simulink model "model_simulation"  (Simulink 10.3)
settings: Solver=VariableStepDiscrete  StartTime=0.0  StopTime=ts  RelTol=1e-3  EnableMultiTasking=on
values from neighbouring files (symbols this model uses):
  A = [0.9944 -0.1203 -0.4302    [model.m]
  Ao1 = A - K1*c1    [model.m]
  Ao2 = A - K2*c2    [model.m]
  Ao3 = A - K3*c3    [model.m]
  B = [0.4252 -0.0082 0.1813]'    [model.m]
  Bo1 = [B K1]    [model.m]
  Bo2 = [B K2]    [model.m]
  Bo3 = [B K3]    [model.m]
  C = eye(3)    [model.m]
  Co1 = c1    [model.m]
  Co2 = c2    [model.m]
  Co3 = c3    [model.m]
  D = zeros(3,1)    [model.m]
  Do1 = zeros(1,2)    [model.m]
  Do2 = zeros(1,2)    [model.m]
  Do3 = zeros(1,2)    [model.m]
  Tc = 0.1    [model.m]
  tf1 = ts/2    (= 25)    [model.m]
  tf2 = ts/2    (= 25)    [model.m]
  tf3 = ts/2    (= 25)    [model.m]
  x0 = [0.05 0.15 0.2]    [model.m]

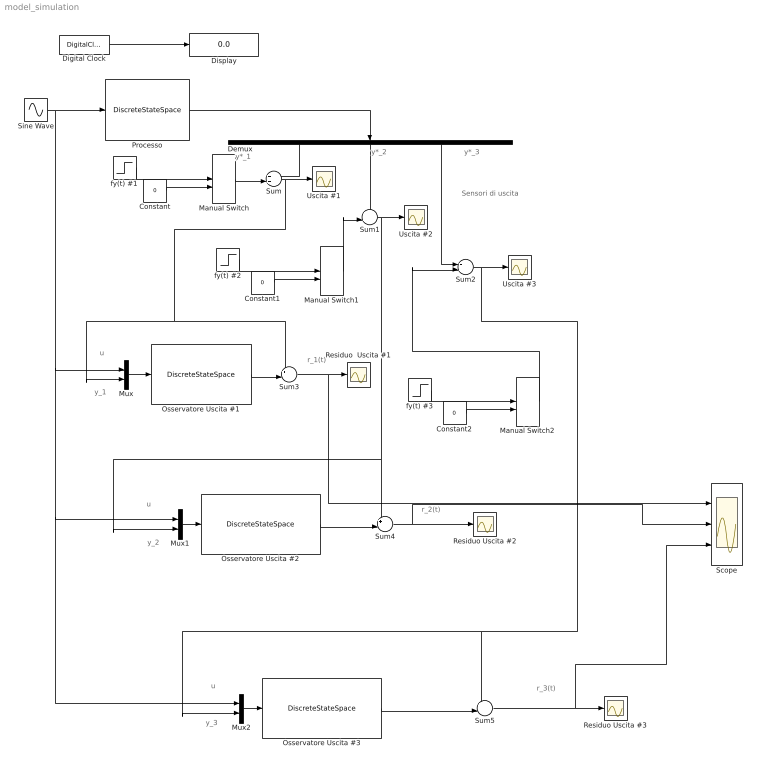
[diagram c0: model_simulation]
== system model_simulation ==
  note: Sensori di uscita
  note: y*_3
  note: y*_2
  note: y*_1
  note: u
  note: y_1
  note: u
  note: y_2
  note: u
  note: y_3
  note: r_1(t)
  note: r_2(t)
  note: r_3(t)
  Constant : Constant  Value=0
  Constant1 : Constant  Value=0
  Constant2 : Constant  Value=0
  Demux : Demux  Outputs=3
  Digital Clock : DigitalClock  SampleTime=0.1
  Display : Display
  Manual Switch : ManualSwitch  CurrentSetting=0
  Manual Switch1 : ManualSwitch
  Manual Switch2 : ManualSwitch  CurrentSetting=0
  Mux : Mux  Inputs=2
  Mux1 : Mux  Inputs=2
  Mux2 : Mux  Inputs=2
  Osservatore Uscita #1 : DiscreteStateSpace  A=Ao1  B=Bo1  C=Co1  D=Do1  SampleTime=Tc
  Osservatore Uscita #2 : DiscreteStateSpace  A=Ao2  B=Bo2  C=Co2  D=Do2  SampleTime=Tc
  Osservatore Uscita #3 : DiscreteStateSpace  A=Ao3  B=Bo3  C=Co3  D=Do3  SampleTime=Tc
  Processo : DiscreteStateSpace  A=A  B=B  C=C  D=D  InitialCondition=x0  SampleTime=Tc
  Residuo Uscita #2 : Scope
  Residuo Uscita #3 : Scope
  Residuo  Uscita #1 : Scope
  Scope : Scope  NumInputPorts=3
  Sine Wave : Sin  SampleTime=Tc
  Sum : Sum  Inputs=++|  SaturateOnIntegerOverflow=on
  Sum1 : Sum  Inputs=++|  SaturateOnIntegerOverflow=on
  Sum2 : Sum  Inputs=++|  SaturateOnIntegerOverflow=on
  Sum3 : Sum  Inputs=+-|  SaturateOnIntegerOverflow=on
  Sum4 : Sum  Inputs=+-|  SaturateOnIntegerOverflow=on
  Sum5 : Sum  Inputs=+-|  SaturateOnIntegerOverflow=on
  Uscita #1 : Scope
  Uscita #2 : Scope
  Uscita #3 : Scope
  fy(t) #1 : Step  Time=tf1  SampleTime=Tc
  fy(t) #2 : Step  Time=tf2  SampleTime=Tc
  fy(t) #3 : Step  Time=tf3  SampleTime=Tc
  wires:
  Sine Wave/1 -> Processo/1, Mux/1, Mux1/1, Mux2/1
  Processo/1 -> Demux/1
  Osservatore Uscita #1/1 -> Sum3/2
  Mux/1 -> Osservatore Uscita #1/1
  Demux/1 -> Sum/1
  Demux/2 -> Sum1/1
  Demux/3 -> Sum2/1
  Digital Clock/1 -> Display/1
  Sum/1 -> Uscita #1/1, Mux/2, Sum3/1
  Sum1/1 -> Uscita #2/1, Mux1/2, Sum4/1
  Sum2/1 -> Uscita #3/1, Mux2/2, Sum5/1
  Sum3/1 -> Scope/1, Residuo  Uscita #1/1
  Osservatore Uscita #2/1 -> Sum4/2
  Mux1/1 -> Osservatore Uscita #2/1
  Sum4/1 -> Scope/2, Residuo Uscita #2/1
  Osservatore Uscita #3/1 -> Sum5/2
  Mux2/1 -> Osservatore Uscita #3/1
  Sum5/1 -> Scope/3, Residuo Uscita #3/1
  fy(t) #1/1 -> Manual Switch/1
  Manual Switch/1 -> Sum/2
  Constant/1 -> Manual Switch/2
  fy(t) #2/1 -> Manual Switch1/1
  Constant1/1 -> Manual Switch1/2
  Manual Switch1/1 -> Sum1/2
  fy(t) #3/1 -> Manual Switch2/1
  Constant2/1 -> Manual Switch2/2
  Manual Switch2/1 -> Sum2/2
